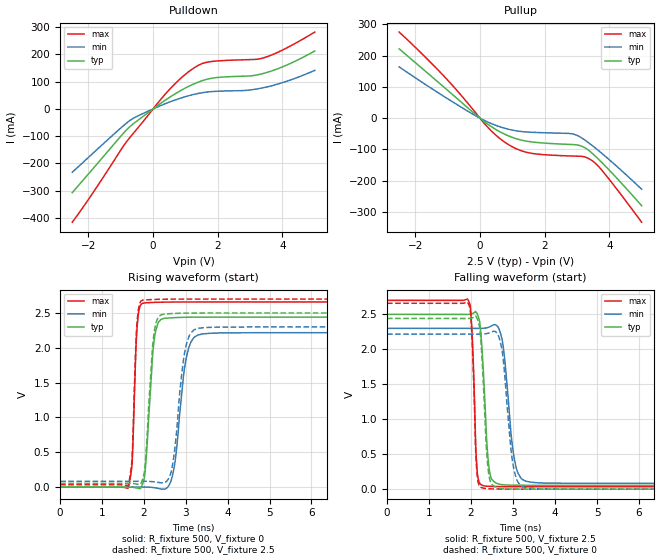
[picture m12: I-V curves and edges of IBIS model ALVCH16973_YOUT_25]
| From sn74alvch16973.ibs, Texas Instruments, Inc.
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[Model]   ALVCH16973_YOUT_25
Model_type  Output
Vref =   0
Rref =   500
Cref =   30p
Vmeas =   1.25
| variable   typ   min   max
C_comp   4.03pF   2.85pF   5.18pF
| C_pullup   4.13pF   3.17pF   4.65pF
| C_pulldown   3.92pF   2.85pF   5.18pF
[Temperature Range]   40   100   -40
| Ambient temperature   25   85   -40
[Voltage range]   2.5   2.3   2.7
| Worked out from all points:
|   slope of the pulldown table from 0 to 0.375 V, typ, clamps not added: 11.7 ohm
|   slope of the pullup table from 0 to 0.375 V, typ, clamps not added: 13.2 ohm
|   rising waveform, R_fixture 500, V_fixture 0: 20-80 % time 153ps typ, 227ps min, 88.6ps max; typ from 0 V to 2.44 V
|   falling waveform, R_fixture 500, V_fixture 2.5: 20-80 % time 130ps typ, 205ps min, 85.6ps max; typ from 2.5 V to 0.055 V
|   rising waveform, R_fixture 500, V_fixture 2.5: 20-80 % time 150ps typ, 219ps min, 87.4ps max; typ from 0.055 V to 2.5 V
|   falling waveform, R_fixture 500, V_fixture 0: 20-80 % time 124ps typ, 197ps min, 86.3ps max; typ from 2.44 V to 0 V
[Pulldown]
| ALVCH16973_YOUT_25
|   Voltage   I(typ)   I(min)   I(max)
-2.5V     -306.8mA   -232.3mA   -415.4mA
-1.855V   -218.5mA   -161.9mA   -306.5mA
-920mV    -89.45mA   -61.74mA   -136.6mA
-675mV    -60.54mA   -39.01mA   -98.65mA
400mV     34mA       20.24mA    57.53mA
1.06V     80.47mA    47.19mA    132.8mA
1.405V    98.7mA     57.06mA    160.3mA
1.675V    109.1mA    62.08mA    171.6mA
2.865V    120.3mA    68.04mA    180.6mA
3.45V     131.5mA    78.9mA     188.7mA
4.15V     161.9mA    102.3mA    224.9mA
5V        212.6mA    141.5mA    281.9mA
[Pullup]
| ALVCH16973_YOUT_25
|   Voltage   I(typ)   I(min)   I(max)
-2.5V     222mA      164.2mA    275.6mA
-1.26V    112.3mA    79.27mA    150.4mA
-295mV    25.76mA    17.27mA    37.77mA
220mV     -17.49mA   -11.3mA    -26.61mA
635mV     -44.4mA    -28.19mA   -66.72mA
1.05V     -63.22mA   -39.15mA   -94.25mA
1.465V    -73.95mA   -44.3mA    -109.8mA
2.85V     -84.33mA   -50.02mA   -121.1mA
3.145V    -89.72mA   -63.15mA   -122.2mA
3.4V      -106.1mA   -81.89mA   -131.5mA
3.83V     -148.2mA   -117.9mA   -174.2mA
5V        -280.1mA   -227.4mA   -332.9mA
[Ramp]
| ALVCH16973_YOUT_25
| variable   typ   min   max
dV/dt_r   1.48/1.70E-10   1.35/2.41E-10   1.60/9.55E-11
dV/dt_f   1.49/1.45E-10   1.36/2.26E-10   1.61/9.34E-11
R_load = 500
[Rising Waveform]
| ALVCH16973_YOUT_25
R_fixture =   500
C_fixture =   0
L_fixture =   0
V_fixture =   0
V_fixture_min = 0
V_fixture_max = 0
|   Time   V(typ)   V(min)   V(max)
0s        6.47nV     29.37nV    168pV
1.62ns    861.8uV    47.07uV    -16.32mV
1.72ns    -1.109mV   153.4uV    354.2mV
1.845ns   -14.52mV   482.4uV    2.349V
2.01ns    134.1mV    1.461mV    2.645V
2.245ns   2.108V     -7.306mV   2.652V
2.485ns   2.424V     -28.98mV   2.656V
3.035ns   2.439V     1.917V     2.658V
3.41ns    2.441V     2.2V       2.658V
29.99ns   2.441V     2.217V     2.659V
[Falling Waveform]
| ALVCH16973_YOUT_25
R_fixture =   500
C_fixture =   0
L_fixture =   0
V_fixture =   2.5
V_fixture_min = 2.3
V_fixture_max = 2.7
|   Time   V(typ)   V(min)   V(max)
0s        2.5V       2.3V       2.7V
1.94ns    2.5V       2.3V       2.695V
2.025ns   2.508V     2.299V     2.227V
2.15ns    2.502V     2.299V     239mV
2.34ns    1.125V     2.304V     44.35mV
2.49ns    143.7mV    2.336V     39.13mV
2.75ns    64.01mV    2.107V     36.56mV
3.075ns   56.65mV    309.8mV    35.28mV
3.415ns   55.44mV    100mV      34.97mV
29.99ns   54.93mV    83.57mV    34.87mV
[Rising Waveform]
| ALVCH16973_YOUT_25
R_fixture =   500
C_fixture =   0
L_fixture =   0
V_fixture =   2.5
V_fixture_min = 2.3
V_fixture_max = 2.7
|   Time   V(typ)   V(min)   V(max)
0s        54.93mV    83.57mV    34.87mV
1.62ns    55.69mV    83.62mV    20.48mV
1.72ns    53.75mV    83.71mV    423.5mV
1.84ns    42.5mV     83.96mV    2.391V
1.98ns    136.1mV    84.6mV     2.687V
2.235ns   2.171V     77.18mV    2.694V
2.48ns    2.484V     64.37mV    2.698V
3ns       2.498V     2.015V     2.7V
3.32ns    2.499V     2.282V     2.7V
29.99ns   2.5V       2.3V       2.7V
[Falling Waveform]
| ALVCH16973_YOUT_25
R_fixture =   500
C_fixture =   0
L_fixture =   0
V_fixture =   0
V_fixture_min = 0
V_fixture_max = 0
|   Time   V(typ)   V(min)   V(max)
0s        2.441V     2.217V     2.659V
1.93ns    2.441V     2.217V     2.661V
2.015ns   2.447V     2.217V     2.258V
2.145ns   2.439V     2.216V     209.3mV
2.335ns   972.2mV    2.221V     9.886mV
2.485ns   71.72mV    2.246V     4.24mV
2.745ns   8.396mV    1.961V     1.623mV
3.035ns   1.743mV    248.8mV    464.8uV
3.39ns    494.3uV    13.53mV    102.7uV
29.99ns   -628.2pV   19.99nV    -2.756nV
